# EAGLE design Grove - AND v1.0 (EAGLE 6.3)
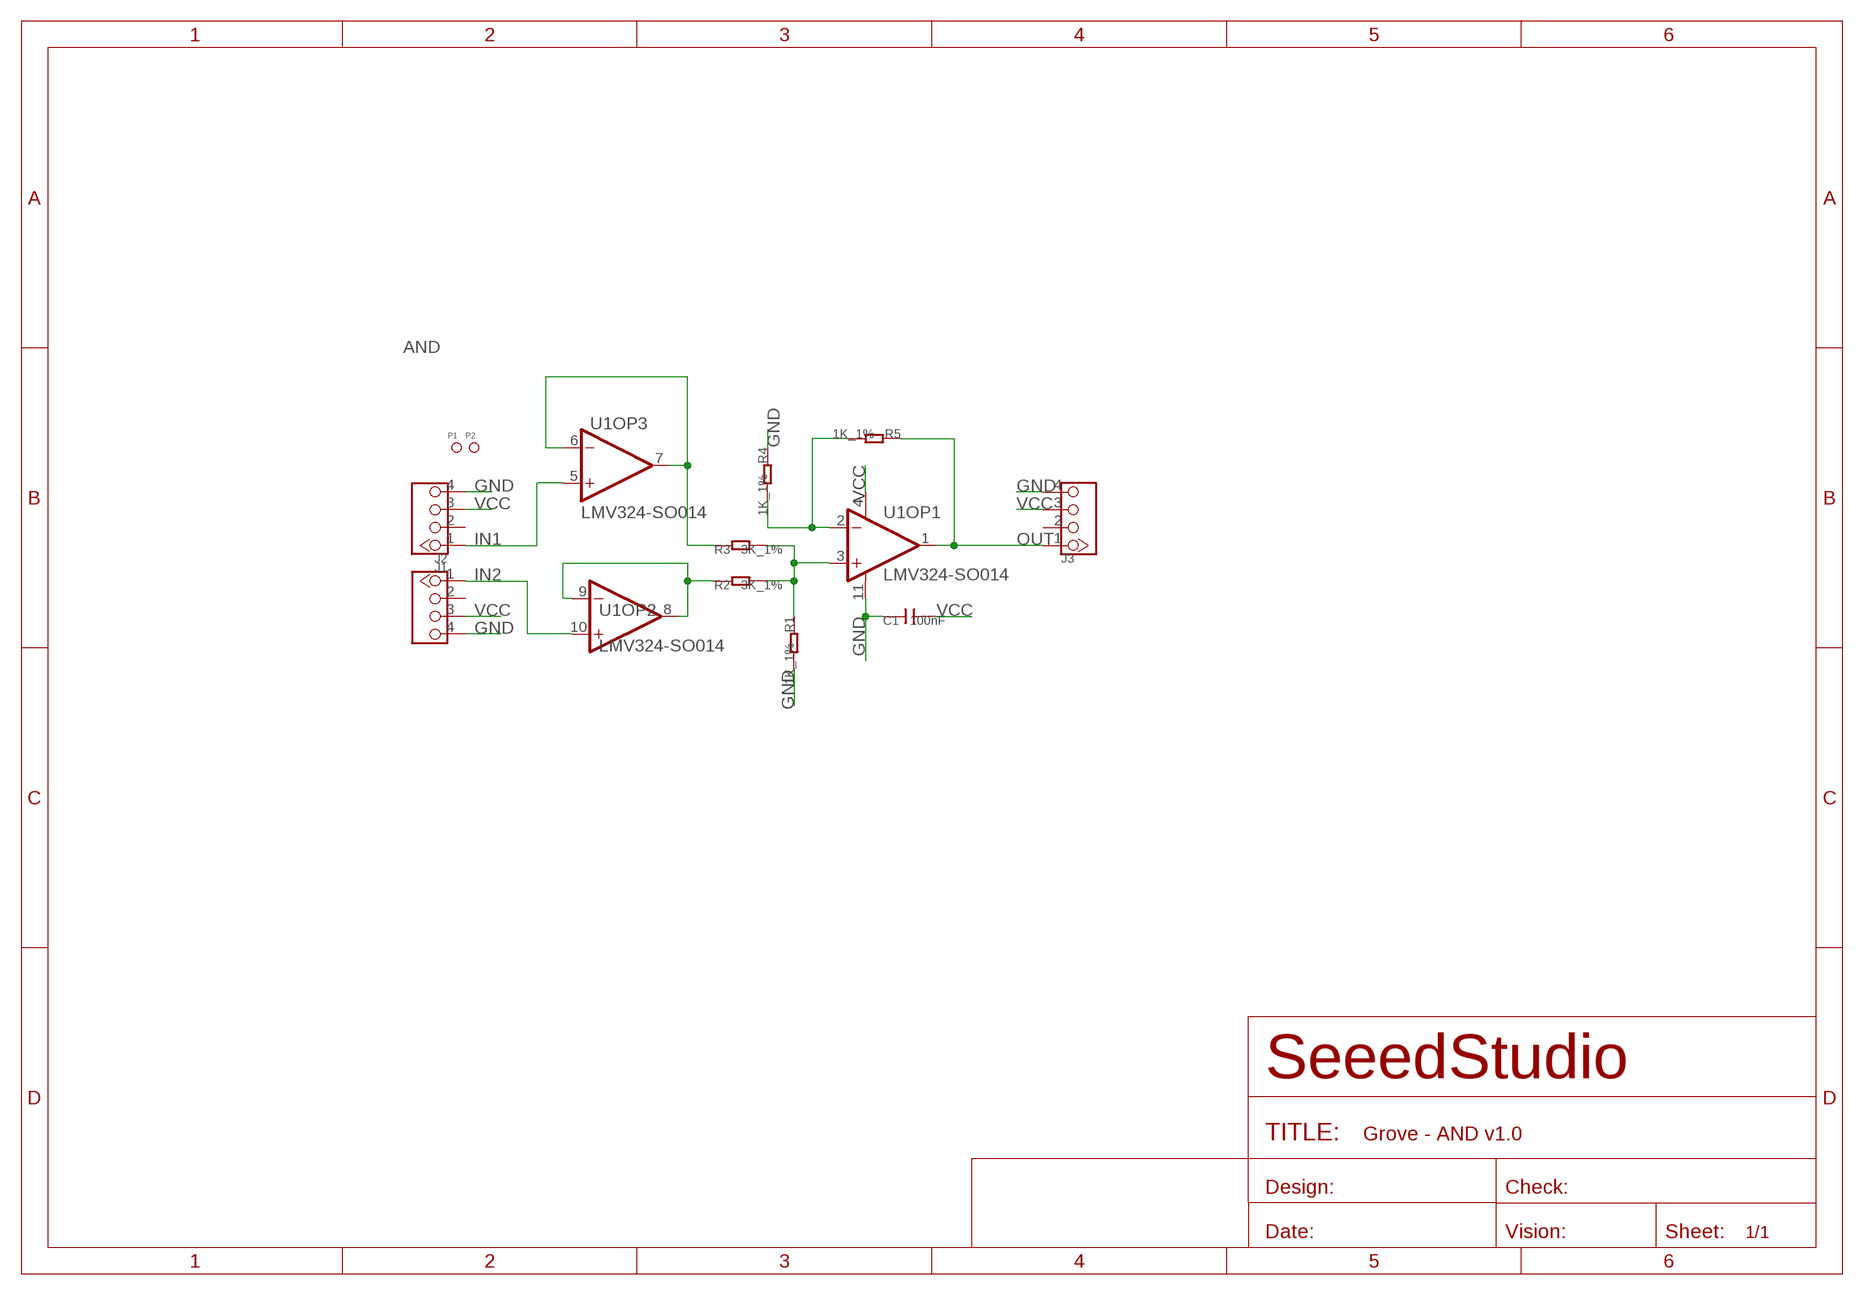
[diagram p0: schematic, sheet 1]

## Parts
C1  100nF  C-0603  [C0603]
J1  TWIG-4P-2.0'90D'  [4P-2.0-90D]
J2  TWIG-4P-2.0'90D'  [4P-2.0-90D]
J3  TWIG-4P-2.0'90D'  [4P-2.0-90D]
P1  PAD-MARK  [ROUND-MARK-1.0]
P2  PAD-MARK  [ROUND-MARK-1.0]
R1  1K_1%  R-0603  [R0603]
R2  3K_1%  R-0603  [R0603]
R3  3K_1%  R-0603  [R0603]
R4  1K_1%  R-0603  [R0603]
R5  1K_1%  R-0603  [R0603]
U1  LMV324-SO014  [SO014]

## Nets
GND: C1.1 J1.4 J2.4 J3.4 R1.2 R4.1 U1.11(OP1:V-)
IN1: J2.1 U1.5(OP3:IN+)
IN2: J1.1 U1.10(OP2:IN+)
N$8: R1.1 R2.2 R3.2 U1.3(OP1:IN+)
N$9: R4.2 R5.2 U1.2(OP1:IN-)
N$12: R2.1 U1.8(OP2:OUT) U1.9(OP2:IN-)
N$15: R3.1 U1.6(OP3:IN-) U1.7(OP3:OUT)
OUT: J3.1 R5.1 U1.1(OP1:OUT)
VCC: C1.2 J1.3 J2.3 J3.3 U1.4(OP1:V+)
Unconnected: J1.2 J2.2 J3.2 U1.12(OP4:IN+) U1.13(OP4:IN-) U1.14(OP4:OUT)

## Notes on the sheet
- AND

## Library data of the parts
C1 = Discrete:C*: Ceramic Capacitors
J1-J3 = Connector:TWIG-4P-2.0
P1 P2 = Discrete:PAD-MARK; PARTNO: DNP
R1-R5 = Discrete:R*
U1 = IC:LMV324: General purpose LOW Voltage, Rail-to-Rail Output Amplifiers http://www.fairchildsemi.com/ds/LM/LMV358.pdf

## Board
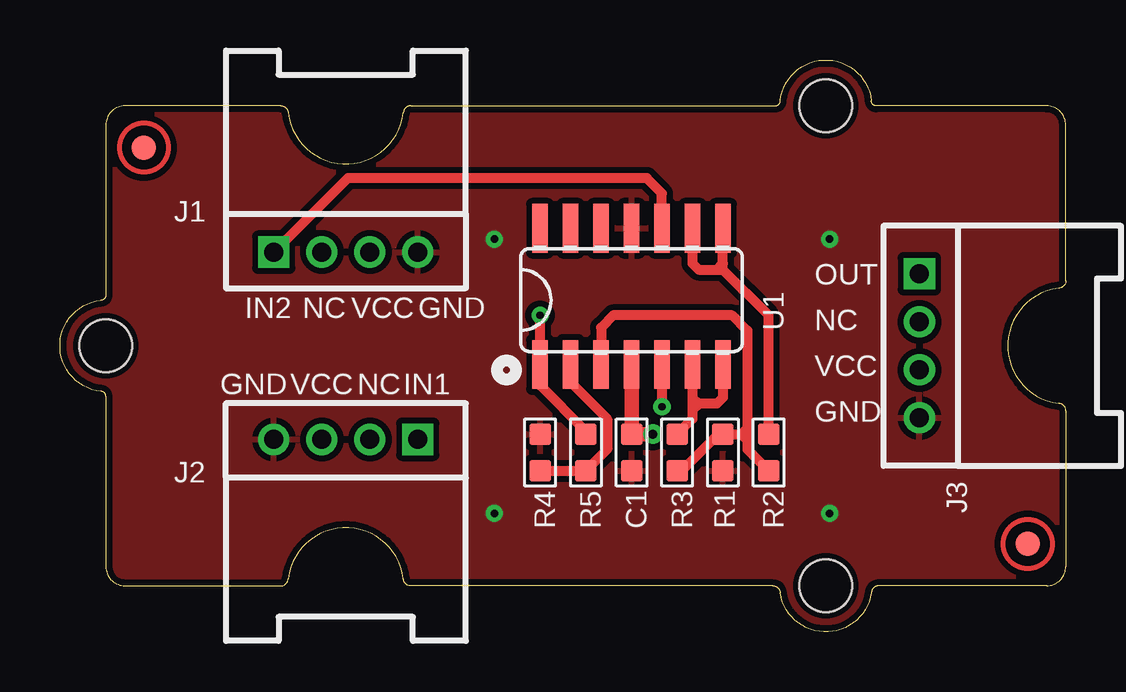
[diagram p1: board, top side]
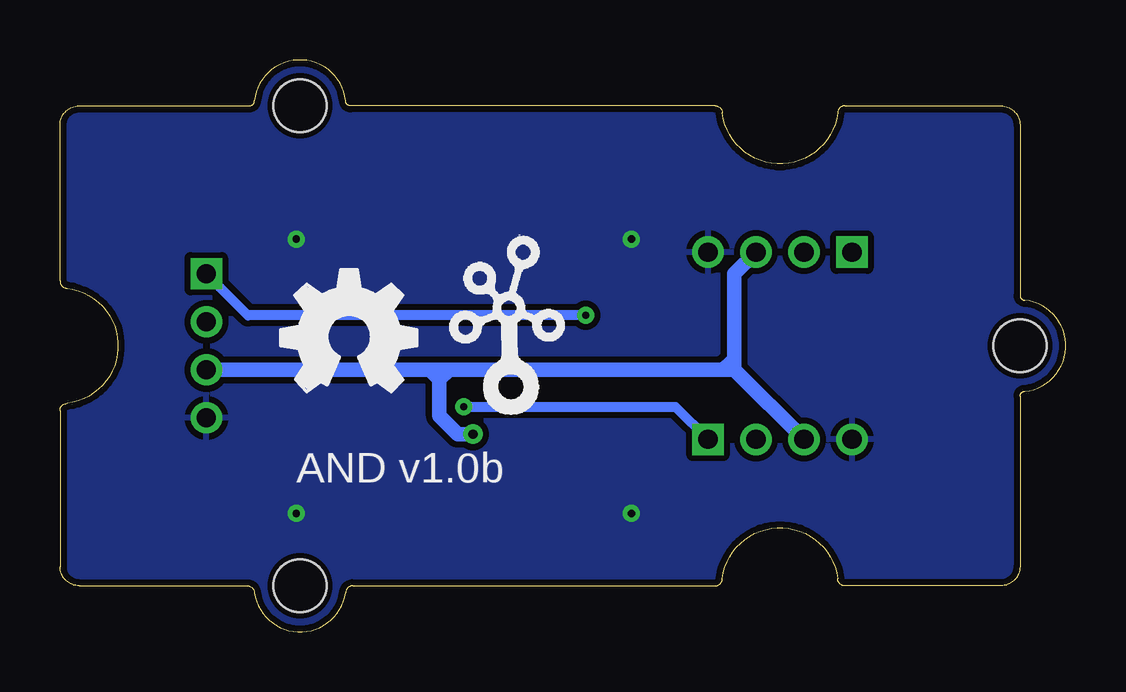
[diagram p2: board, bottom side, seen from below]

Size 41.91 x 23.83 mm. Coordinates in mm from the lower left corner, seen from the top.
Copper layers (1*16): Top 0.035mm / dielectric 1.5mm / Bottom 0.035mm
Design rules "default *": minimum track width 10mil, minimum drill 10mil, track to track 6mil, track to pad 6mil, pad to pad 6mil, via to via 6mil, smd to smd 0mil, copper to edge 10mil, drill to drill 8mil, minimum pad ring 10mil, minimum via ring 8mil, stop-mask expansion 4mil, vias tented up to drill 100mil, thermal gap 10mil

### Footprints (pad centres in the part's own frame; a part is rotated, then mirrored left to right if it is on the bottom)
C0603 = smd 0.889 x 0.889: 1 -0.762,0; 2 0.762,0
4P-2.0-90D = drill 0.8 pad 1.27 square: 1 -3,0 | drill 0.8 pad 1.27: 2 -1,0; 3 1,0; 4 3,0
ROUND-MARK-1.0 = smd 1.016 x 1.016: P$1 0,0
R0603 = smd 0.889 x 0.889: 1 -0.762,0; 2 0.762,0
SO014 = smd 0.66 x 2.032: 1 -3.175,-2.68; 2 -1.905,-2.68; 3 -0.635,-2.68; 4 0.635,-2.68; 5 1.905,-2.68; 6 3.175,-2.68; 7 4.445,-2.68; 8 4.445,2.997; 9 3.175,2.997; 10 1.905,2.997; 11 0.635,2.997; 12 -0.635,2.997; 13 -1.905,2.997; 14 -3.175,2.997
2U-DIM-W/DRILL = hole 2.2: -10,-10; -10,10; 20,0

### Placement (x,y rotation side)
C1  23.81,7.48 90 top
J1  11.91,15.82 0 top
J2  11.91,8.02 180 top
J3  35.81,11.92 270 top
P1  3.49,20.18 0 top
P2  40.32,3.67 0 top
R1  27.62,7.48 270 top
R2  29.53,7.48 270 top
R3  25.72,7.48 270 top
R4  20,7.48 270 top
R5  21.91,7.48 270 top
U1  23.18,13.83 0 top
U$1  [2U-DIM-W/DRILL]  21.91,11.92 180 top
U$2  [OSHW_FILLX200_NOTEXT]  32.7,10.02 0 bottom
U$5  [TWIGLOGO]  23.18,10.02 0 bottom

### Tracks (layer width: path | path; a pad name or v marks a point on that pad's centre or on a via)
GND  (via drill 0.3 pad 0.64)
  other vias: 18.1,16.37 18.1,4.94 32.07,16.37 32.07,4.94
  pour Bottom (isolate 0.254): -0.32,-0.14 42.23,-0.14 42.23,23.99 -0.32,23.99
  pour Top (isolate 0.254): -0.32,-0.14 42.23,-0.14 42.23,23.99 -0.32,23.99
IN1  (via drill 0.3 pad 0.64)
  Top 0.406: U1.5 v25.08,9.38
  Bottom 0.406: v25.08,9.38 16.27,9.38 J2.1
IN2
  Top 0.406: U1.10 25.08,18.27 24.45,18.91 11.99,18.91 J1.1
N$8
  Top 0.406: U1.3 22.54,12.68 23.05,13.19 28,13.19 28.64,12.56 28.64,8.49 | 28.64,8.49 28.64,8.11 | 28.64,8.11 28.64,7.98 | 28.64,7.98 28.64,7.6 R2.2 | 28.39,8.24 R1.1 27.43,8.24 25.91,6.71 R3.2 | 28.39,8.24 28.51,8.24 28.64,8.11 | 28.39,8.24 28.64,8.49 | 28.39,8.24 28.64,7.98
N$9
  Top 0.406: U1.2 21.27,10.4 22.8,8.87 22.8,7.6 R5.2 R4.2
N$12
  Top 0.406: R2.1 29.53,13.19 27.62,15.1 | 27.62,15.1 27.62,15.35 | 27.62,15.35 U1.8 | U1.9 26.35,15.35 26.61,15.1 27.37,15.1 | 27.37,15.1 27.62,15.1 | 27.37,15.1 27.62,15.35
N$15
  Top 0.406: U1.6 26.35,9.76 | 26.35,9.76 26.35,9.64 | 26.35,9.64 26.35,9.51 | 26.35,9.51 26.35,9.25 | 26.35,9.25 26.35,8.87 R3.1 | U1.7 27.62,9.76 27.37,9.51 26.61,9.51 | 26.48,9.51 26.35,9.51 | 26.61,9.51 26.48,9.51 | 26.48,9.51 26.35,9.64 | 26.61,9.51 26.35,9.76 | 26.61,9.51 26.35,9.25
OUT  (via drill 0.3 pad 0.64)
  Top 0.406: R5.1 21.91,8.37 20,10.27 U1.1 v20,13.19
  Bottom 0.406: v20,13.19 34.08,13.19 J3.1
VCC  (via drill 0.38 pad 0.81)
  Top 0.61: U1.4 C1.2 v24.7,8.24
  Bottom 0.61: J3.3 25.97,10.92 | 25.97,10.92 14.27,10.92 | 14.27,10.92 13.81,10.92 | 13.81,10.92 J2.3 | 13.81,10.92 13.81,14.92 J1.3 | 14.27,10.92 13.91,11.29 | v24.7,8.24 25.34,8.24 26.1,9 26.1,10.52 | 26.1,10.52 26.1,10.79 25.97,10.92 | 26.1,10.52 25.72,10.91 | 26.1,10.52 26.48,10.91

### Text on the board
tPlace: OUT | IN2 | NC | VCC | GND | NC | VCC | GND | VCC | NC | IN1 | GND
bPlace: AND v1.0b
